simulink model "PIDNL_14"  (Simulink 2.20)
settings: Solver=VariableStepDiscrete  StartTime=0.0  StopTime=40.0  RelTol=1e-3  AbsTol=1e-6
undefined symbols (not defined in the file or in its folder): fnl, pidin
libraries: simulink x3, Puma x2

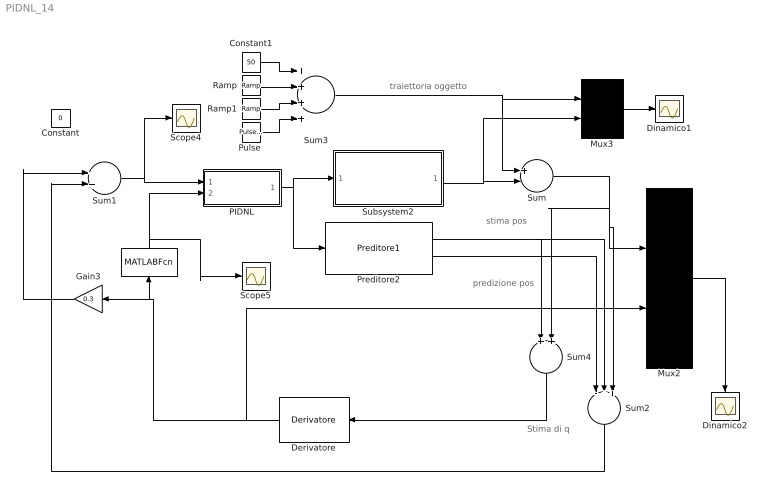
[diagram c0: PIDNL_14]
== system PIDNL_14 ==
  note: traiettoria oggetto
  note: stima pos
  note: predizione pos
  note: Stima di q
  " " : MATLABFcn  Orientation=up  MATLABFcn=fnl(u(1))  OutputWidth=-1
  Constant : Constant  Value=0
  Constant1 : Constant  Value=50
  Derivatore : Puma/Derivatore  Orientation=left  Td=0.13  T=0.033  N=3
  Dinamico1 : Scope
  Dinamico2 : Scope
  Gain3 : Gain  Orientation=left  Gain=0.3
  Mux2 : Mux  Inputs=2
  Mux3 : Mux  Inputs=2
  PIDNL : Subsystem
  Preditore2 : Puma/Preditore1  Ts=.260
  "Pulse " : simulink/Sources/Pulse Generator  period=30  duty=10  amplitude=-50  start=30
  Ramp : simulink/Sources/Ramp  slope=-50  start=10  X0=0
  Ramp1 : simulink/Sources/Ramp  slope=+50  start=25  X0=0
  Scope4 : Scope
  Scope5 : Scope
  Subsystem2 : Subsystem  mask(Modello del Puma 260 in Alter Mode){Ts=.260}
      mask prompts: Ts "Tempo di Campionamento Ts della seriale"
      mask help: Questo blocco racchiude il comportamento dinamico del Puma 260 pilotato dalla seriale. La rappresentazione e' a variabili di stato.
      mask init:
      | K=10; % attenuazione del guadagno puma.
      | A=[0,0,0,0,0,0,0,0,0,0;
      | 1,0,0,0,0,0,0,0,0,0;
      | 0,1,0,0,0,0,0,0,0,0;
      | 0,0,1,0,0,0,0,0,0,0;
      | 0,0,0,1,0,0,0,0,0,0;
      | 0,0,0,0,1,0,0,0,0,0;
      | 0,0,0,0,0,1,0,0,0,0;
      | 0,0,0,0,0,0,1,0,0,0;
      | 0,0,0,0,0,0,0,1,0,0;
      | 0,0,0,0,0,0,0,0,1/K,1];
      | B=[1;0;0;0;0;0;0;0;0;0];
      | C=[0,0,0,0,0,0,0,0,0,1];
      | D=[0];
  Sum : Sum  Inputs=+-
  Sum1 : Sum  Inputs=++
  Sum2 : Sum  Orientation=down  Inputs=-++
  Sum3 : Sum  Inputs=++++
  Sum4 : Sum  Orientation=down  Inputs=++
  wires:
  Mux2/1 -> Dinamico2/1
  Subsystem2/1(Out1) -> Sum/2, Mux3/2
  Mux3/1 -> Dinamico1/1
  Sum3/1 -> Sum/1, Mux3/1
  Sum2/1 -> Sum1/2
  Constant1/1 -> Sum3/1
  Ramp/1 -> Sum3/2
  Ramp1/1 -> Sum3/3
  Sum4/1 -> Derivatore/1
  Sum/1 -> Mux2/1, Sum2/3, Sum4/2
  PIDNL/1(Out1) -> Preditore2/1, Subsystem2/1(In1)
  Sum1/1 -> Scope4/1, PIDNL/1(In1)
  " "/1 -> Scope5/1, PIDNL/2(In2)
  Preditore2/1 -> Sum2/2, Sum4/1
  Preditore2/2 -> Sum2/1
  Gain3/1 -> Sum1/1
  "Pulse "/1 -> Sum3/4
  Derivatore/1 -> " "/1, Gain3/1, Mux2/2

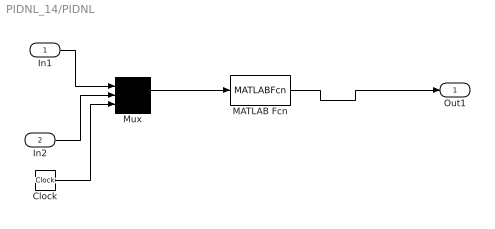
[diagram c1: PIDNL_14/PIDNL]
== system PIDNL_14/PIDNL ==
  In1 : Inport  Port=1  PortWidth=-1  SampleTime=-1
  In2 : Inport  Port=2  PortWidth=-1  SampleTime=-1
  Clock : Clock
  MATLAB Fcn : MATLABFcn  MATLABFcn=pidin(u(1),u(2),u(3))  OutputWidth=1
  Mux : Mux  Inputs=3
  Out1 : Outport  Port=1
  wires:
  MATLAB Fcn/1 -> Out1/1
  Mux/1 -> MATLAB Fcn/1
  In1/1 -> Mux/1
  In2/1 -> Mux/2
  Clock/1 -> Mux/3

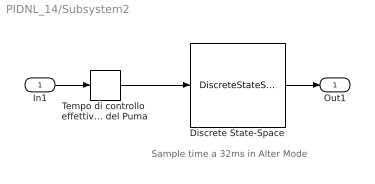
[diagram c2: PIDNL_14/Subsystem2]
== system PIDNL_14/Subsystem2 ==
  note: Sample time a 32ms in Alter Mode
  In1 : Inport  Port=1  PortWidth=-1  SampleTime=-1
  Discrete State-Space : DiscreteStateSpace  A=A  B=B  C=C  D=D  X0=0  SampleTime=.032
  Tempo di controllo  effettivo Ts del Puma : ZeroOrderHold  SampleTime=Ts
  Out1 : Outport  Port=1
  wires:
  In1/1 -> Tempo di controllo  effettivo Ts del Puma/1
  Discrete State-Space/1 -> Out1/1
  Tempo di controllo  effettivo Ts del Puma/1 -> Discrete State-Space/1
